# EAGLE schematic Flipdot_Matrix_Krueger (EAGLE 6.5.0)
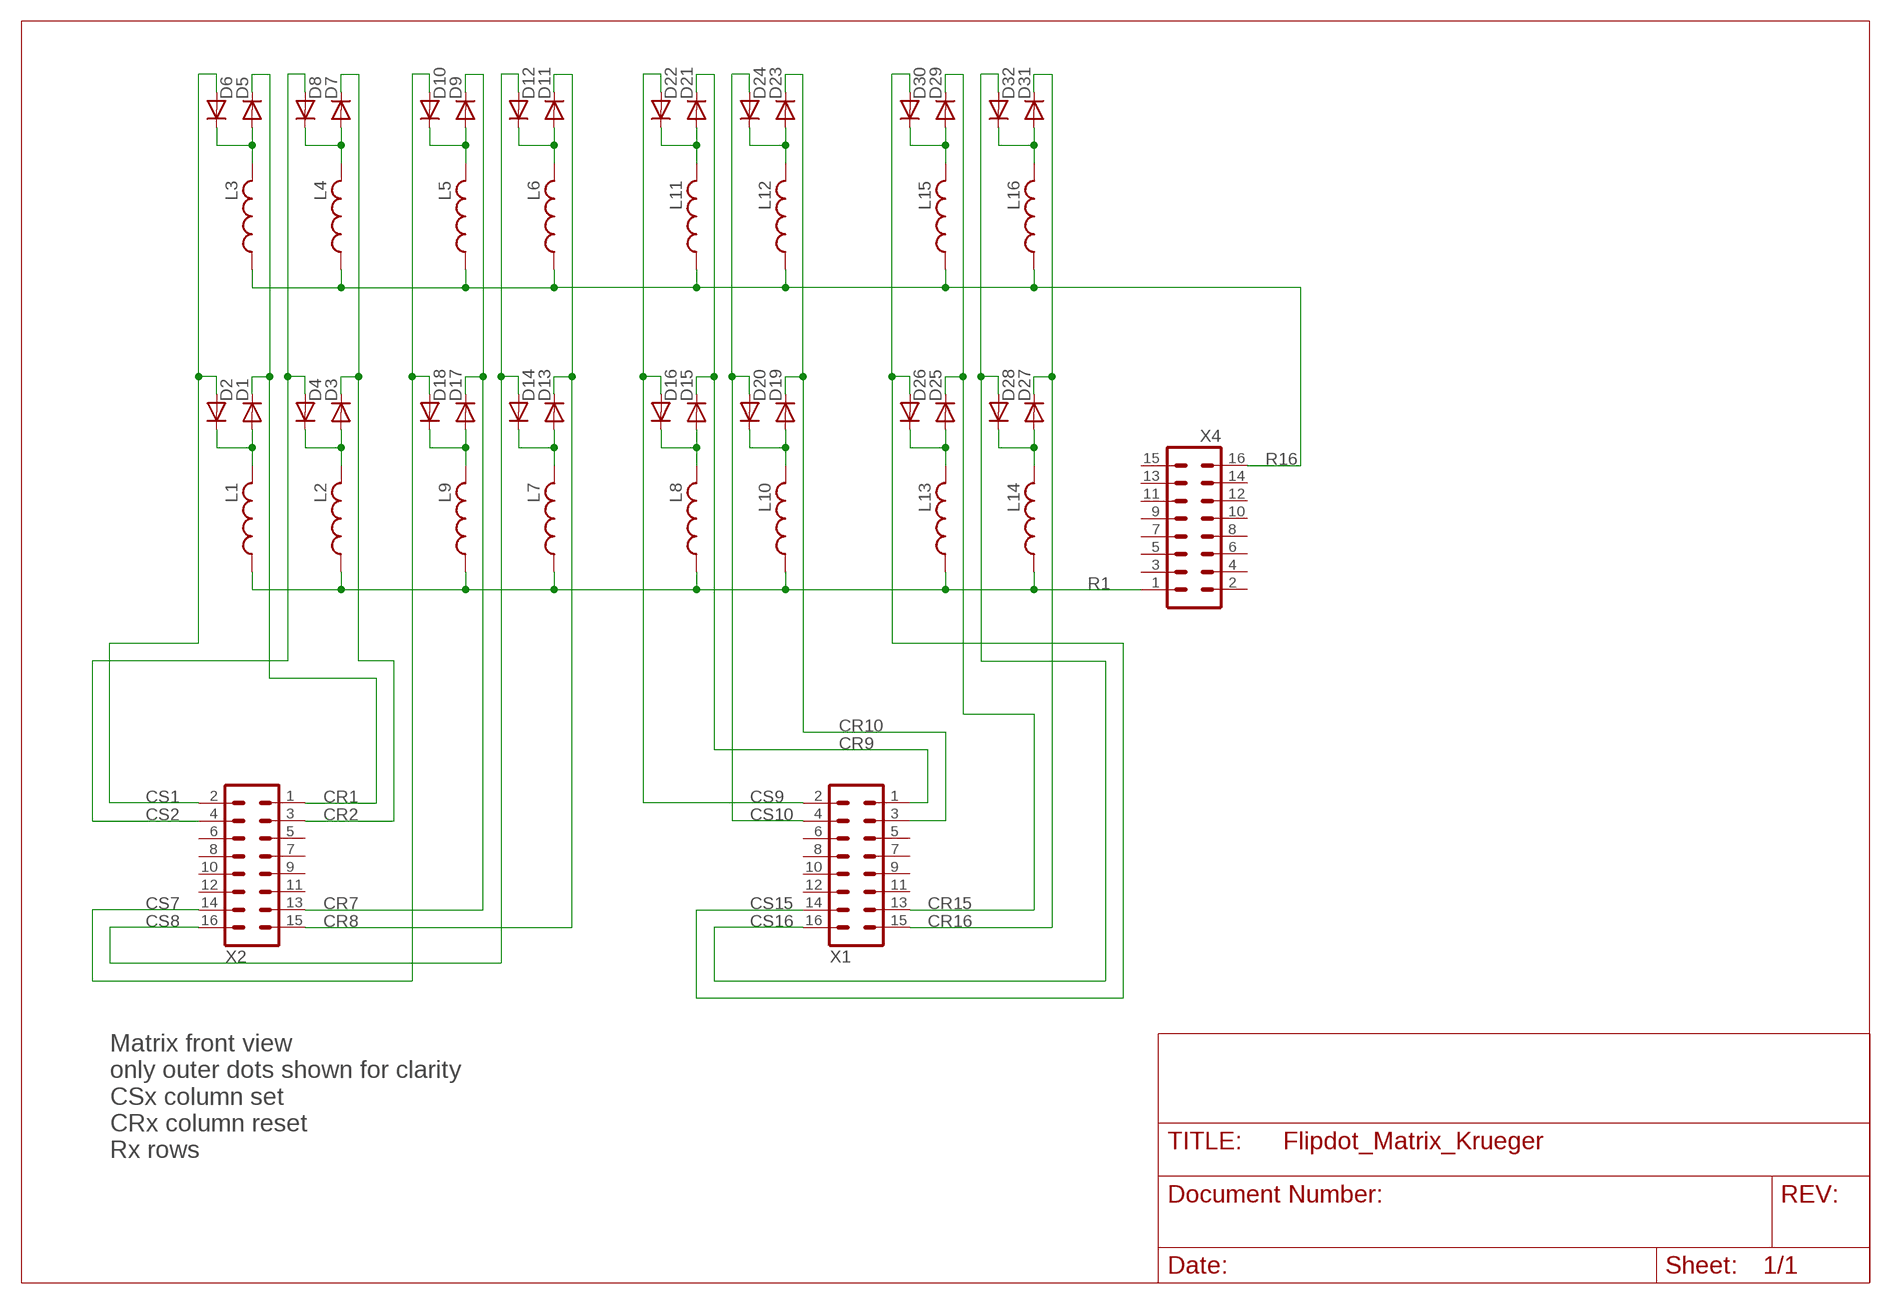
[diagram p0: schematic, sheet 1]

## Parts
D1  1N4004  [DO41-10]
D2  1N4004  [DO41-10]
D3  1N4004  [DO41-10]
D4  1N4004  [DO41-10]
D5  1N4004  [DO41-10]
D6  1N4004  [DO41-10]
D7  1N4004  [DO41-10]
D8  1N4004  [DO41-10]
D9  1N4004  [DO41-10]
D10  1N4004  [DO41-10]
D11  1N4004  [DO41-10]
D12  1N4004  [DO41-10]
D13  1N4004  [DO41-10]
D14  1N4004  [DO41-10]
D15  1N4004  [DO41-10]
D16  1N4004  [DO41-10]
D17  1N4004  [DO41-10]
D18  1N4004  [DO41-10]
D19  1N4004  [DO41-10]
D20  1N4004  [DO41-10]
D21  1N4004  [DO41-10]
D22  1N4004  [DO41-10]
D23  1N4004  [DO41-10]
D24  1N4004  [DO41-10]
D25  1N4004  [DO41-10]
D26  1N4004  [DO41-10]
D27  1N4004  [DO41-10]
D28  1N4004  [DO41-10]
D29  1N4004  [DO41-10]
D30  1N4004  [DO41-10]
D31  1N4004  [DO41-10]
D32  1N4004  [DO41-10]
L1  L-US0204V  [0204V]
L2  L-US0204V  [0204V]
L3  L-US0204V  [0204V]
L4  L-US0204V  [0204V]
L5  L-US0204V  [0204V]
L6  L-US0204V  [0204V]
L7  L-US0204V  [0204V]
L8  L-US0204V  [0204V]
L9  L-US0204V  [0204V]
L10  L-US0204V  [0204V]
L11  L-US0204V  [0204V]
L12  L-US0204V  [0204V]
L13  L-US0204V  [0204V]
L14  L-US0204V  [0204V]
L15  L-US0204V  [0204V]
L16  L-US0204V  [0204V]
X1  MA08-2  [MA08-2]
X2  MA08-2  [MA08-2]
X4  ML16  [ML16]

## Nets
CR1: D1.C D5.C X2.1
CR2: D3.C D7.C X2.3
CR7: D9.C D17.C X2.13
CR8: D11.C D13.C X2.15
CR9: D15.C D21.C X1.1
CR10: D19.C D23.C X1.3
CR15: D25.C D29.C X1.13
CR16: D27.C D31.C X1.15
CS1: D2.A D6.A X2.2
CS2: D4.A D8.A X2.4
CS7: D10.A D18.A X2.14
CS8: D12.A D14.A X2.16
CS9: D16.A D22.A X1.2
CS10: D20.A D24.A X1.4
CS15: D26.A D30.A X1.14
CS16: D28.A D32.A X1.16
N$1: D7.A D8.C L4.2
N$2: D1.A D2.C L1.2
N$3: D3.A D4.C L2.2
N$4: D9.A D10.C L5.2
N$5: D5.A D6.C L3.2
N$6: D11.A D12.C L6.2
N$7: D13.A D14.C L7.2
N$8: D15.A D16.C L8.2
N$9: D17.A D18.C L9.2
N$10: D19.A D20.C L10.2
N$15: D21.A D22.C L11.2
N$16: D23.A D24.C L12.2
N$21: D25.A D26.C L13.2
N$22: D27.A D28.C L14.2
N$27: D29.A D30.C L15.2
N$28: D31.A D32.C L16.2
R1: L1.1 L2.1 L7.1 L8.1 L9.1 L10.1 L13.1 L14.1 X4.1
R16: L3.1 L4.1 L5.1 L6.1 L11.1 L12.1 L15.1 L16.1 X4.16
Unconnected: X1.5 X1.6 X1.7 X1.8 X1.9 X1.10 X1.11 X1.12 X2.5 X2.6 X2.7 X2.8 X2.9 X2.10 X2.11 X2.12 X4.2 X4.3 X4.4 X4.5 X4.6 X4.7 X4.8 X4.9 X4.10 X4.11 X4.12 X4.13 X4.14 X4.15

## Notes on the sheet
- Matrix front view
  only outer dots shown for clarity
  CSx column set
  CRx column reset
  Rx rows

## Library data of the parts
D1-D32 = diode:1N4004: DIODE
L1-L16 = rcl:L-US: INDUCTOR, American symbol
X1 X2 = con-lstb:MA08-2: PIN HEADER; OC_FARNELL: unknown; OC_NEWARK: unknown
X4 = con-harting-ml:ML16: HARTING; OC_FARNELL: unknown; OC_NEWARK: unknown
